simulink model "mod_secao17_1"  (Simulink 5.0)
settings: Solver=ode45  StartTime=0.0  StopTime=0.0016  MaxStep=0.0000001  RelTol=1e-6

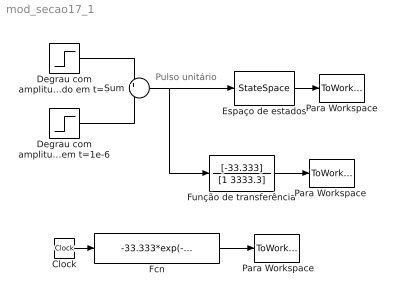
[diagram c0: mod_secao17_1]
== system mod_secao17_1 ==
  note: Pulso unitário
  " Para Workspace" : ToWorkspace  VariableName=V3_an  SampleTime=-1  SaveFormat=Array
  Clock : Clock
  Degrau com amplitude 1e6 aplicado em t=0 : Step  Time=0  After=1e6  SampleTime=0
  Degrau com amplitude 1e6 aplicado em t=1e-6 : Step  Time=1e-6  After=1e6  SampleTime=0
  Espaço de estados : StateSpace  A=-3333.3  B=0  D=0  X0=-33.333
  Fcn : Fcn  Expr=-33.333*exp(-3333.3*u)
  Função de transferência : TransferFcn  Numerator=[-33.333]  Denominator=[1 3333.3]
  Para Workspace : ToWorkspace  VariableName=V3_ss  SampleTime=-1  SaveFormat=Array
  "Para Workspace " : ToWorkspace  VariableName=V3_tf  SampleTime=-1  SaveFormat=Array
  Sum : Sum  Inputs=+-
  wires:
  Sum/1 -> Espaço de estados/1, Função de transferência/1
  Degrau com amplitude 1e6 aplicado em t=0/1 -> Sum/1
  Degrau com amplitude 1e6 aplicado em t=1e-6/1 -> Sum/2
  Espaço de estados/1 -> Para Workspace/1
  Função de transferência/1 -> "Para Workspace "/1
  Clock/1 -> Fcn/1
  Fcn/1 -> " Para Workspace"/1
